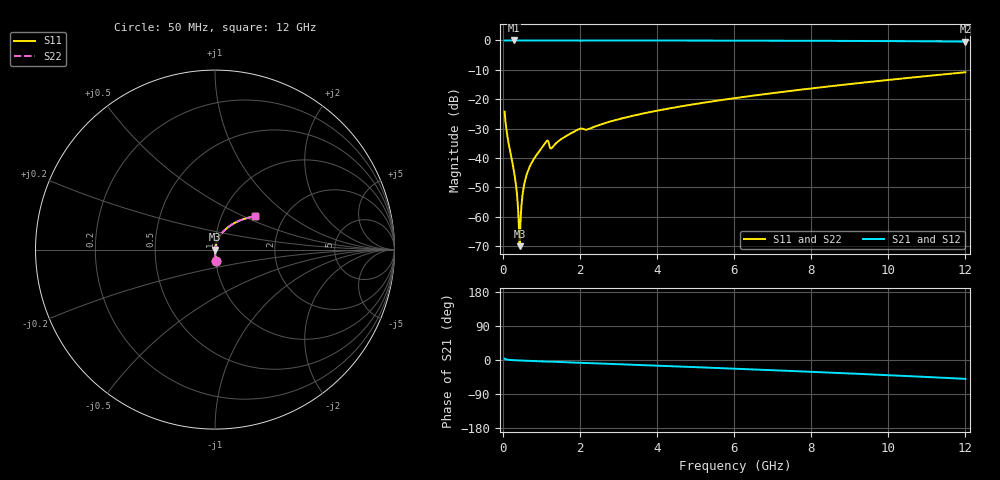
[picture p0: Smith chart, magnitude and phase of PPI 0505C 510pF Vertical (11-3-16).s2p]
# GHz S MA R 50
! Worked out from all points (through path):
!   1601 points, 50 MHz to 12 GHz, reference 50 ohm
!   highest |S21| = 0.00 dB at 281.5 MHz (marker M1); lowest = -0.4 dB at 12 GHz (marker M2)
!   group delay of S21, straight-line fit = 11.5 ps
!   lowest |S11| = -70.0 dB at 438.4 MHz (marker M3), VSWR 1.00, Z = 50 - j0.000972 ohm
!   |S11| at or under -10 dB: start of sweep to end of sweep
!   |S22| runs from -70.0 to -10.8 dB; largest |S21 - S12| = 0
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0.05  0.06142 -86.5  0.9979 3.4  0.9979 3.4  0.06142 -86.5
0.1545625  0.01767 -88.7  0.9996 0.6  0.9996 0.6  0.01767 -88.7
0.2815313  0.006531 -88.0  0.9997 -0.4  0.9997 -0.4  0.006531 -88.0
0.3412812  0.003627 -86.2  0.9997 -0.8  0.9997 -0.8  0.003627 -86.2
0.4010313  0.001314 -77.6  0.9997 -1.1  0.9997 -1.1  0.001314 -77.6
0.438375  0.0003159 -1.8  0.9997 -1.2  0.9997 -1.2  0.0003159 -1.8
0.4757188  0.001216 73.1  0.9996 -1.4  0.9996 -1.4  0.001216 73.1
0.5354688  0.002915 81.6  0.9996 -1.7  0.9996 -1.7  0.002915 81.6
0.6026875  0.004688 83.7  0.9996 -2.0  0.9996 -2.0  0.004688 83.7
0.7147187  0.007424 84.5  0.9995 -2.5  0.9995 -2.5  0.007424 84.5
0.8715625  0.0111 84.4  0.9994 -3.1  0.9994 -3.1  0.0111 84.4
1.1255  0.01884 76.7  0.9968 -4.3  0.9968 -4.3  0.01884 76.7
1.282344  0.01501 74.9  0.997 -4.5  0.997 -4.5  0.01501 74.9
1.596031  0.02258 81.9  0.9987 -5.8  0.9987 -5.8  0.02258 81.9
2.044156  0.03163 74.6  0.9951 -7.6  0.9951 -7.6  0.03163 74.6
2.208469  0.03078 76.0  0.9962 -8.0  0.9962 -8.0  0.03078 76.0
2.962813  0.04486 77.9  0.9979 -11.0  0.9979 -11.0  0.04486 77.9
4.038312  0.06442 74.1  0.9968 -15.1  0.9968 -15.1  0.06442 74.1
6.025  0.1044 66.5  0.9932 -22.9  0.9932 -22.9  0.1044 66.5
8.019156  0.153 58.4  0.9866 -31.2  0.9866 -31.2  0.153 58.4
10.01331  0.2132 49.5  0.975 -40.1  0.975 -40.1  0.2132 49.5
12  0.2875 39.9  0.9554 -49.8  0.9554 -49.8  0.2875 39.9
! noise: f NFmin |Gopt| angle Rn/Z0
0.05  0.000295  0.8249  0.2075  0.0003541
1.372  0.004386  0.6993  3.829  0.002851
2.701  0.005431  0.5614  7.259  0.002218
4.031  0.006256  0.4676  10.27  0.001971
5.36  0.007584  0.4324  13.16  0.002179
6.682  0.008962  0.4128  15.86  0.002444
8.012  0.01041  0.4025  18.43  0.002753
9.341  0.01194  0.3995  20.89  0.003118
10.67  0.0136  0.4028  23.27  0.003554
12  0.01542  0.4118  25.64  0.004087
